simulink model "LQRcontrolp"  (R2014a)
settings: Solver=ode4  StartTime=0.0  StopTime=2  FixedStep=t0  RelTol=1e-3
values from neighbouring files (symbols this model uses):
  k1 = k(1)    [LQRposition.m]    (also in LQRvelocity.m)
  k2 = k(2)    [LQRposition.m]    (also in LQRvelocity.m)
  t0 = 0.0002    [LQRposition.m]    (also in LQRvelocity.m)
undefined symbols (not defined in the file or in its folder): ae, be, ce, de
libraries: xpcnilib x3, slrtlib x3, simulink x1, powerlib_meascontrol x1

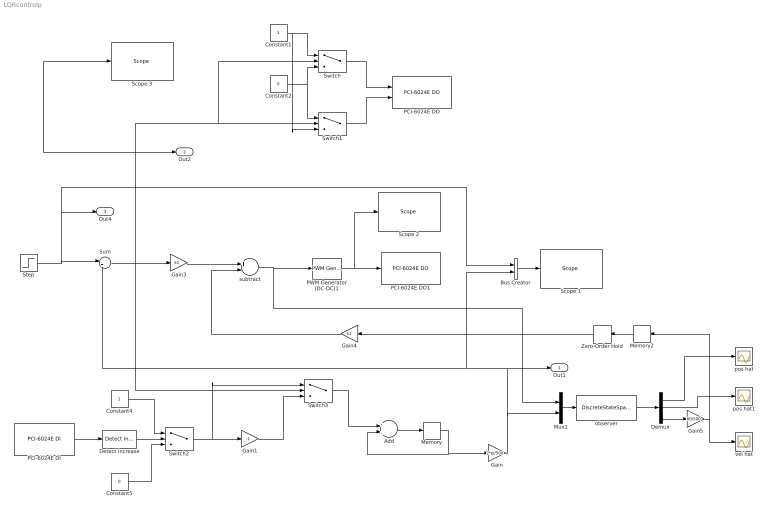
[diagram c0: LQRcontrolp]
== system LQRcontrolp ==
  Add : Sum
  Bus Creator : BusCreator  Inputs=2
  Constant1 : Constant
  Constant2 : Constant  Value=0
  Constant4 : Constant
  Constant5 : Constant  Value=0
  Demux : Demux  Outputs=3
  Detect Increase : simulink/Logic and Bit Operations/Detect Increase  vinit=0.0  InputProcessing=Inherited  OutDataTypeStr=boolean
  Gain : Gain  Gain=2*pi/500
  Gain1 : Gain  Gain=-1
  Gain3 : Gain  Gain=k1
  Gain4 : Gain  Gain=k2
  Gain5 : Gain  Gain=60/500
  Memory : Memory  InheritSampleTime=on
  Memory2 : Memory
  Mux1 : Mux  Inputs=2
  PCI-6024E DI : xpcnilib/Digital Input/E Series/PCI-6024E DI  channel=[4]  sampletime=t0  slot=-1
  PCI-6024E DO : xpcnilib/Digital Output/E Series/PCI-6024E DO  channel=[1 2]  reset=[1]  initValue=[0]  sampletime=-1  slot=-1
  PCI-6024E DO1 : xpcnilib/Digital Output/E Series/PCI-6024E DO  channel=[3]  reset=[1]  initValue=[0]  sampletime=-1  slot=-1
  PWM Generator (DC-DC)1 : powerlib_meascontrol/Pulse & Signal Generators/PWM Generator (DC-DC)  Fsw=1000  Ts=t0
  Scope 1 : slrtlib/Displays and Logging/Scope   scopeno=1  scopetype=Target  autostart=on  viewmode=Graphical redraw  formatstr='%15.6f'  grid=on  ylimits=[0,0]  nosamples=2000  noprepostsamples=0  interleave=1  triggermode=FreeRun  triggersignal=1  trigsignalfromport=off  triggerlevel=0.0  triggerslope=Either  triggerscope=1  triggersample=0  filename=data.dat  mode=Lazy  writesize=512  autorestart=off  dynamicfilemode=off  maxwritefilesize=512*1024^2
  Scope 2 : slrtlib/Displays and Logging/Scope   scopeno=3  scopetype=Target  autostart=on  viewmode=Graphical redraw  formatstr='%15.6f'  grid=on  ylimits=[0,0]  nosamples=2000  noprepostsamples=0  interleave=1  triggermode=FreeRun  triggersignal=1  trigsignalfromport=off  triggerlevel=0.0  triggerslope=Either  triggerscope=1  triggersample=0  filename=data.dat  mode=Lazy  writesize=512  autorestart=off  dynamicfilemode=off  maxwritefilesize=512*1024^2
  Scope 3 : slrtlib/Displays and Logging/Scope   scopeno=2  scopetype=Target  autostart=on  viewmode=Graphical redraw  formatstr='%15.6f'  grid=on  ylimits=[0,0]  nosamples=2000  noprepostsamples=0  interleave=1  triggermode=FreeRun  triggersignal=1  trigsignalfromport=off  triggerlevel=0.0  triggerslope=Either  triggerscope=1  triggersample=0  filename=data.dat  mode=Lazy  writesize=512  autorestart=off  dynamicfilemode=off  maxwritefilesize=512*1024^2
  Step : Step  Time=0.2  After=2  SampleTime=t0
  Sum : Sum  Inputs=|+-
  Switch{,1..3} (4 alike) : Switch  Criteria=u2 > Threshold
  Zero-Order Hold : ZeroOrderHold  SampleTime=t0
  observer : DiscreteStateSpace  A=ae  B=be  C=ce  D=de  X0=[0 0]  SampleTime=t0
  pos hat : Scope
  pos hat1 : Scope
  subtract : Sum  Inputs=+-
  vel hat : Scope
  Out1 : Outport
  Out2 : Outport  Port=2
  Out4 : Outport  Port=3
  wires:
  Gain/1 -> Mux1/2, Bus Creator/2, Sum/2, Out1/1
  Constant1/1 -> Switch1/3, Switch/1
  Constant2/1 -> Switch1/1, Switch/3
  Switch/1 -> PCI-6024E DO/1
  Switch1/1 -> PCI-6024E DO/2
  Add/1 -> Memory/1
  Memory/1 -> Add/2, Gain/1
  PCI-6024E DI/1 -> Detect Increase/1
  Sum/1 -> Gain3/1, Switch3/2, Scope 3/1, Switch/2, Switch1/2, Out2/1
  Detect Increase/1 -> Switch2/2
  Constant4/1 -> Switch2/1
  Constant5/1 -> Switch2/3
  Step/1 -> Bus Creator/1, Out4/1, Sum/1
  Switch2/1 -> Gain1/1, Switch3/1
  Switch3/1 -> Add/1
  Gain1/1 -> Switch3/3
  PWM Generator (DC-DC)1/1 -> PCI-6024E DO1/1, Scope 2/1
  Gain4/1 -> subtract/2
  Gain3/1 -> subtract/1
  subtract/1 -> PWM Generator (DC-DC)1/1, Mux1/1
  Bus Creator/1 -> Scope 1/1
  Mux1/1 -> observer/1
  observer/1 -> Demux/1
  Demux/3 -> Gain5/1
  Memory2/1 -> Zero-Order Hold/1
  Zero-Order Hold/1 -> Gain4/1
  Demux/1 -> pos hat/1
  Demux/2 -> pos hat1/1
  Gain5/1 -> vel hat/1, Memory2/1
